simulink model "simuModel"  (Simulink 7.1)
settings: Solver=VariableStepDiscrete  StartTime=0.0  StopTime=100  RelTol=1e-3
undefined symbols (not defined in the file or in its folder): gray
libraries: vipsnks x2, dspsrcs4 x1

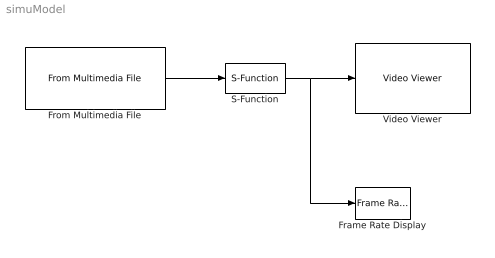
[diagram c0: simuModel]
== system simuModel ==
  Frame Rate Display : vipsnks/Frame Rate Display  DialogController=vipDDGCreate  DialogControllerArgs=DataTag0  UpdateRate=10
  From Multimedia File : dspsrcs4/From Multimedia File  DialogController=dspDDGCreate  DialogControllerArgs=DataTag1  inputFilename=vipmen.avi  loop=on  numPlays=inf  outputStreams=Video only  videoDataType=uint8  audioDataType=int16  inheritSampleTime=off  userDefinedSampleTime=1/30  noAudioOutput=off  isIntensityVideo=on  colorVideoFormat=One multidimensional signal  outputEOF=off  dataOrg=Column-major
  S-Function : S-Function  FunctionName=simuCuda  EnableBusSupport=off
  Video Viewer : vipsnks/Video Viewer  DialogController=vipDDGCreate  DialogControllerArgs=DataTag2  inputType=Obsolete7b  imagePorts=One multidimensional signal  useColorMap=off  colormapValue=gray(256)  specRange=off  minInputVal=0  maxInputVal=255  FigPos=[880 417 160 128]  AxisZoom=on  trueSizedOnce=on
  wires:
  From Multimedia File/1 -> S-Function/1
  S-Function/1 -> Video Viewer/1, Frame Rate Display/1
